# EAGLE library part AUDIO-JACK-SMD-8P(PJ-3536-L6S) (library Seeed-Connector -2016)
320040003
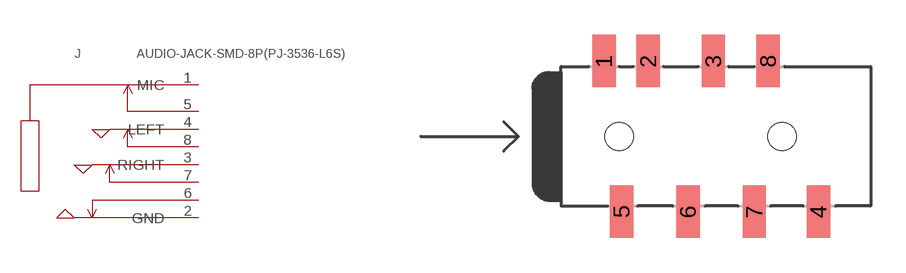
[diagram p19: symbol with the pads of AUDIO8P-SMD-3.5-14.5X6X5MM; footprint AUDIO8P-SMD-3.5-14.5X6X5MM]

Designator prefix J

## AUDIO-JACK-SMD-8P(PJ-3536-L6S) (MPN: PJ-3536-L6S; VALUE: PJ-3536-L6S)  [AUDIO8P-SMD-3.5-14.5X6X5MM]
1  MIC
2  GND
3  RIGHT
4  LEFT
5  5
6  6
7  7
8  8

## Footprint AUDIO8P-SMD-3.5-14.5X6X5MM (pad centres in mm)
smd 1 x 2.25: 1 3.05,3.24; 2 4.95,3.24; 3 7.75,3.24; 4 12.26,-3.24; 5 3.81,-3.24; 6 6.66,-3.24; 7 9.51,-3.24; 8 10.1,3.24
hole 1.2 at 3.7,0
hole 1.2 at 10.7,0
